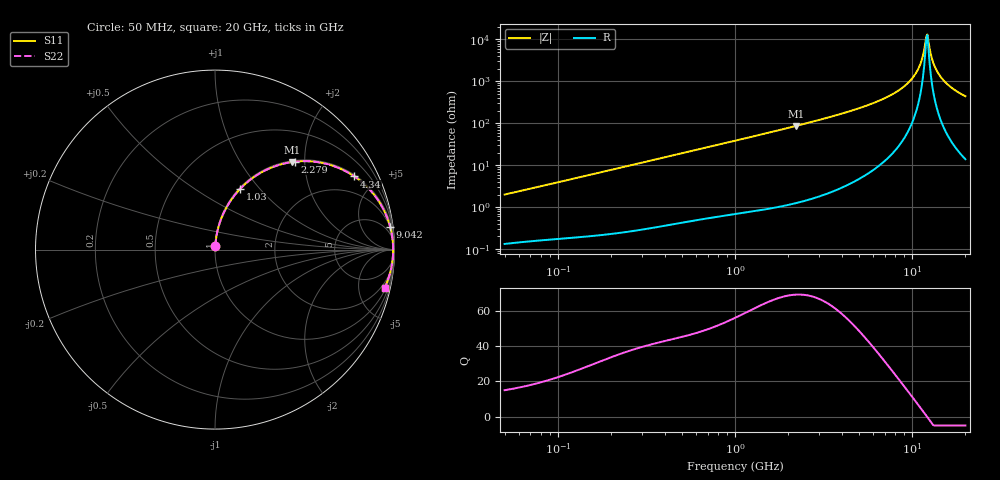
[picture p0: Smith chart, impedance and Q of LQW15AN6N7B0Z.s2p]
!Murata Part Number: LQW15AN6N7B0Z
!These Parameters are Measured in Series Mode Connection
!  o--[Z]--o
!Port1  Port2
!  o-------o
!Freq. Start=50[MHz] Stop=20[GHz], 401[Steps]
# Hz S RI R 50
!Freq.(Hz) S11(Real) S11(Imag) S21(Real) S21(Imag) S12(Real) S12(Imag) S22(Real) S22(Imag)
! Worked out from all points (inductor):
!   401 points, 50 MHz to 20 GHz, reference 50 ohm
!   read as one part in series: L = 6.3 nH near 51.52 MHz
!   highest Q = 69.4 at 2.212 GHz (marker M1), where L = 6.24 nH
!   self-resonance near 12.02 GHz
!   S11 on the Smith chart (normalised r, x): 50 MHz: 1.00, +0.04; 1.03 GHz: 1.01, +0.79; 2.279 GHz: 1.03, +1.79; 4.34 GHz: 1.07, +3.77; 9.042 GHz: 2, +15; 20 GHz: 1.28, -8.84
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5e7  0.00172 0.0199  0.9983 -0.0199  0.9983 -0.0199  0.00172 0.0199
1.364002e8  0.00474 0.0528  0.9953 -0.0528  0.9953 -0.0528  0.00474 0.0528
3.721004e8  0.0234 0.1397  0.9766 -0.1397  0.9766 -0.1397  0.0234 0.1397
1e9  0.1327 0.3304  0.8673 -0.3304  0.8673 -0.3304  0.1327 0.3304
1.030411e9  0.1395 0.3378  0.8605 -0.3378  0.8605 -0.3378  0.1395 0.3378
2.211938e9  0.4305 0.488  0.5695 -0.488  0.5695 -0.488  0.4305 0.488
2.279204e9  0.446 0.4899  0.554 -0.4899  0.554 -0.4899  0.446 0.4899
2.728004e9  0.5419 0.491  0.4581 -0.491  0.4581 -0.491  0.5419 0.491
4.34015e9  0.7761 0.4079  0.2239 -0.4079  0.2239 -0.4079  0.7761 0.4079
7.442007e9  0.9464 0.2081  0.0536 -0.2081  0.0536 -0.2081  0.9464 0.2081
9.041845e9  0.9762 0.1261  0.0238 -0.1261  0.0238 -0.1261  0.9762 0.1261
9.892087e9  0.9847 0.0878  0.0153 -0.0878  0.0153 -0.0878  0.9847 0.0878
1.066139e10  0.9895 0.0558  0.0105 -0.0558  0.0105 -0.0558  0.9895 0.0558
1.131968e10  0.9918 0.0301  0.00824 -0.0301  0.00824 -0.0301  0.9918 0.0301
1.183995e10  0.9926 0.0109  0.00741 -0.0109  0.00741 -0.0109  0.9926 0.0109
1.220001e10  0.9927 -0.00196  0.00728 0.00196  0.00728 0.00196  0.9927 -0.00196
1.238412e10  0.9927 -0.00838  0.00733 0.00838  0.00733 0.00838  0.9927 -0.00838
1.295331e10  0.992 -0.0276  0.00801 0.0276  0.00801 0.0276  0.992 -0.0276
1.334722e10  0.9911 -0.0405  0.00887 0.0405  0.00887 0.0405  0.9911 -0.0405
1.438523e10  0.9875 -0.0725  0.0125 0.0725  0.0125 0.0725  0.9875 -0.0725
1.646126e10  0.9755 -0.1301  0.0245 0.1301  0.0245 0.1301  0.9755 -0.1301
2e10  0.9453 -0.2122  0.0547 0.2122  0.0547 0.2122  0.9453 -0.2122
